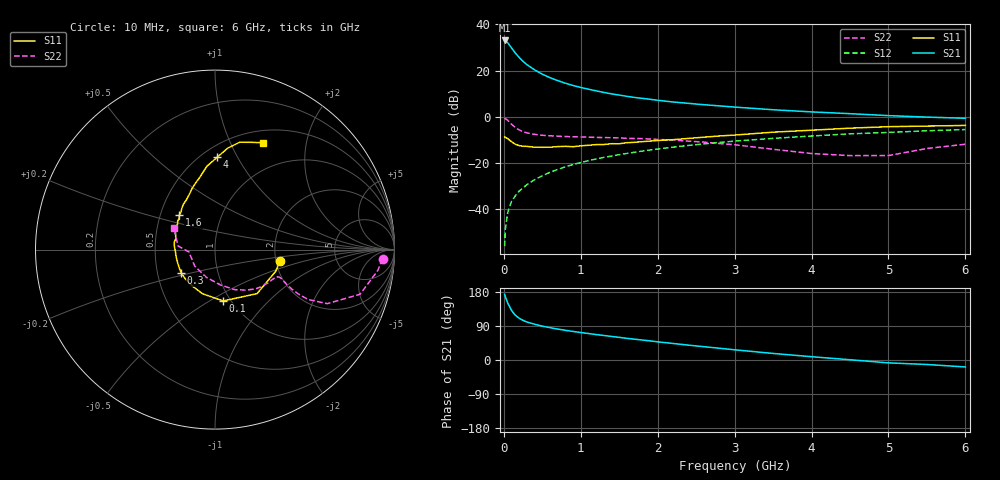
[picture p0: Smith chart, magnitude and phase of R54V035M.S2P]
! SIEMENS Small Signal Semiconductors
! BFR183
! Si NPN RF Bipolar Junction Transistor in SOT23
! VCE = 4 V  IC = 35 mA
! Common Emitter S-Parameters:  May  1996
# GHz  S  MA  R  50
!  f  S11  S21  S12  S22
! GHz  MAG  ANG  MAG  ANG  MAG  ANG  MAG  ANG
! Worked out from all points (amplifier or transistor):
!   36 points, 10 MHz to 6 GHz, reference 50 ohm
!   highest |S21| = 33.1 dB at 10 MHz (marker M1)
!   |S21| within 3 dB of that: start of sweep to 95.01 MHz
!   unconditionally stable (mu >= 1): 406.6 MHz to 2.365 GHz
!   at 250 MHz: K = 0.92, MSG = 27.3 dB, |S12| = -30.7 dB
!   at 1.4 GHz: K = 1.04, MAG = 12.2 dB, |S12| = -16.9 dB
!   at 6 GHz: K = 0.90, MSG = 2.4 dB, |S12| = -5.5 dB
!   S11 on the Smith chart (normalised r, x): 10 MHz: 2.11, -0.31; 100 MHz: 0.92, -0.58; 300 MHz: 0.66, -0.18; 1.6 GHz: 0.63, +0.26; 4 GHz: 0.59, +0.83; 6 GHz: 0.65, +1.34
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0.01  0.3692 -10.0  44.94 173.3  0.0016 91.5  0.9349 -3.2
0.02  0.359 -19.8  44.2 167.0  0.0038 87.3  0.9144 -7.3
0.05  0.3393 -46.3  40.18 150.5  0.0085 76.6  0.8458 -17.1
0.1  0.2897 -81.0  31 130.8  0.0149 71.6  0.6945 -25.7
0.15  0.2554 -105.9  23.97 118.0  0.0197 70.3  0.5873 -28.2
0.2  0.2391 -121.9  19.25 110.2  0.025 72.3  0.5216 -28.0
0.25  0.2324 -134.1  15.85 104.5  0.0292 72.6  0.4783 -27.1
0.3  0.23 -145.0  13.5 100.3  0.0343 73.6  0.4517 -26.2
0.4  0.2212 -159.6  10.38 94.4  0.0438 74.3  0.4186 -24.5
0.5  0.2202 -169.9  8.377 89.4  0.0533 74.4  0.4002 -23.4
0.6  0.2209 -177.6  7.042 85.3  0.0634 74.9  0.3899 -23.2
0.8  0.2306 169.3  5.344 78.4  0.0831 73.5  0.3757 -23.7
0.9  0.2266 164.1  4.772 75.3  0.0935 72.9  0.3712 -24.3
1.1  0.2433 155.1  3.968 69.9  0.1131 71.2  0.364 -26.7
1.3  0.2526 145.6  3.374 64.7  0.1331 69.3  0.3566 -28.9
1.6  0.2764 136.0  2.78 57.1  0.1621 66.0  0.3439 -33.5
2.2  0.3213 119.5  2.1 43.6  0.2216 59.3  0.3148 -44.1
3.5  0.467 95.5  1.426 17.3  0.3429 42.4  0.1992 -81.2
4  0.515 88.6  1.282 8.7  0.3862 36.3  0.1614 -108.0
4.5  0.5701 82.8  1.173 0.7  0.4296 29.5  0.1452 -141.1
5.5  0.6328 70.8  0.989 -11.8  0.5005 17.6  0.207 174.3
6  0.6533 65.6  0.933 -18.4  0.5332 10.0  0.2564 152.7
